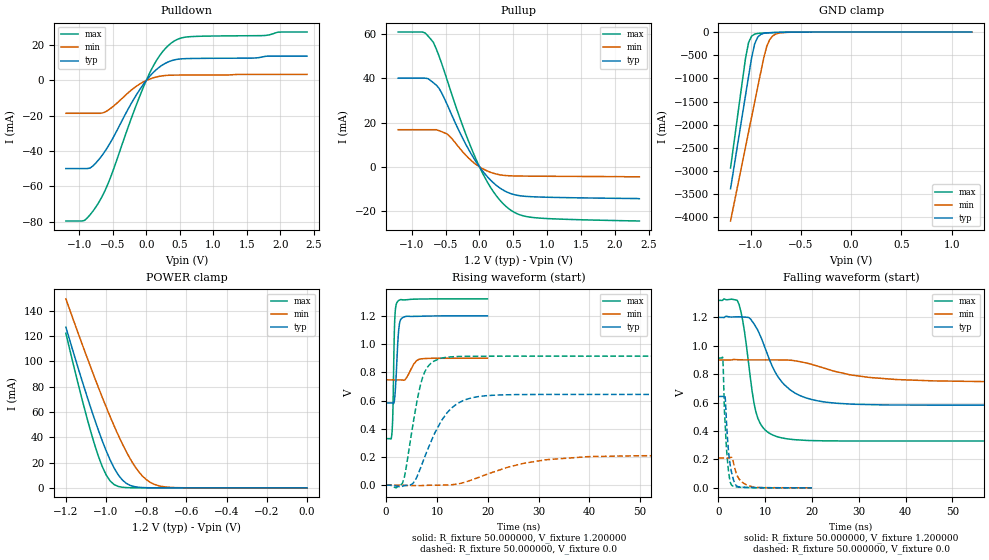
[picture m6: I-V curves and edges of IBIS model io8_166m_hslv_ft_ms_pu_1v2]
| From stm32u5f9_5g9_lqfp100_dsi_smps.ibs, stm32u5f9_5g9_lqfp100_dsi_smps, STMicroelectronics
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|   Model io8_166m_hslv_ft_ms_pu_1v2
[Model]  io8_166m_hslv_ft_ms_pu_1v2
Model_type I/O
Polarity   Non-Inverting
Enable   Active-Low
Vinl =   0.360000V
Vinh =   0.840000V
Vmeas =  0.600000V
Cref =   50.000000pF
Rref =   100.000000M
Vref =   0.0V
C_comp   3.151700pF   3.087200pF   3.197900pF
[Temperature Range]   25.000000   0.140000k   -40.000000
[Pullup Reference]   1.200000V   0.900000V   1.320000V
[Pulldown Reference]   0.0V   0.0V   0.0V
[POWER Clamp Reference]   1.200000V   0.900000V   1.320000V
[GND Clamp Reference]   0.0V   0.0V   0.0V
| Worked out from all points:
|   slope of the pulldown table from 0 to 0.18 V, typ, clamps not added: 25.4 ohm
|   slope of the pullup table from 0 to 0.18 V, typ, clamps not added: 27.8 ohm
|   GND clamp passes 1 mA (typ) near -0.51 V on its own axis
|   POWER clamp passes 1 mA (typ) near -0.86 V on its own axis
|   rising waveform, R_fixture 50.000000, V_fixture 1.200000: 20-80 % time 553ps typ, 1.42ns min, 312ps max; typ from 0.583 V to 1.2 V
|   rising waveform, R_fixture 50.000000, V_fixture 0.0: 20-80 % time 5.19ns typ, 12.1ns min, 2.72ns max; typ from 0 V to 0.643 V
|   falling waveform, R_fixture 50.000000, V_fixture 1.200000: 20-80 % time 5.91ns typ, 12.5ns min, 2.6ns max; typ from 1.2 V to 0.583 V
|   falling waveform, R_fixture 50.000000, V_fixture 0.0: 20-80 % time 1.04ns typ, 1.73ns min, 831ps max; typ from 0.643 V to 0 V
[Pulldown]
|Voltage   I(typ)   I(min)   I(max)
-1.2V     -49.86mA   -18.57mA   -79.56mA
-920mV    -49.86mA   -18.57mA   -79.19mA
-840mV    -49.6mA    -18.57mA   -76.08mA
-720mV    -45.32mA   -18.57mA   -69.74mA
-560mV    -36.71mA   -16.58mA   -57.44mA
-200mV    -11.43mA   -4.74mA    -19.03mA
0V        0A         0A         0A
160mV     6.477mA    2.075mA    11.78mA
360mV     10.99mA    2.99mA     20.81mA
480mV     12.07mA    3.054mA    23.52mA
640mV     12.43mA    3.075mA    24.76mA
2.4V      13.77mA    3.425mA    27.43mA
[Pullup]
|Voltage   I(typ)   I(min)   I(max)
-1.2V     40.07mA    16.78mA    60.91mA
-840mV    40.07mA    16.78mA    60.91mA
-680mV    37.99mA    16.78mA    56.17mA
-600mV    35.62mA    16.38mA    50.27mA
-480mV    28.32mA    14.85mA    39.45mA
-240mV    12.39mA    6.513mA    17.85mA
-40mV     1.772mA    818.2uA    2.67mA
200mV     -7.072mA   -2.851mA   -11mA
440mV     -11.84mA   -4.03mA    -19.1mA
600mV     -13.07mA   -4.154mA   -21.71mA
840mV     -13.59mA   -4.223mA   -23.04mA
2.36V     -14.4mA    -4.5mA     -24.47mA
[GND_clamp]
|Voltage   I(typ)   I(min)   I(max)
-1.2V     -3.379A    -4.076A    -2.932A
-1.05V    -1.35A     -2.47A     -550.7mA
-1.02V    -947.8mA   -2.149A    -221.5mA
-990mV    -552.4mA   -1.829A    -88.44mA
-960mV    -255.3mA   -1.51A     -44.87mA
-930mV    -111.8mA   -1.191A    -30.68mA
-870mV    -28.36mA   -564.6mA   -21.34mA
-840mV    -18.65mA   -309.5mA   -18.49mA
-810mV    -14.07mA   -161.6mA   -15.92mA
-780mV    -11.37mA   -83.33mA   -13.53mA
-600mV    -3.009mA   -4.322mA   -3.091mA
1.2V      0A         13.65nA    0A
[POWER_clamp]
|Voltage   I(typ)   I(min)   I(max)
-1.2V     127mA      149.4mA    122.2mA
-1.12V    84.98mA    114mA      70.29mA
-1.06V    55.52mA    88.42mA    35.69mA
-1.02V    37.64mA    72.04mA    17.19mA
-1V       29.52mA    64.13mA    10.33mA
-960mV    15.7mA     48.99mA    2.596mA
-900mV    3.636mA    28.77mA    207.8uA
-840mV    502.9uA    13.24mA    43.19uA
-800mV    129uA      6.535mA    43.19uA
-740mV    26.51uA    1.726mA    43.19uA
-620mV    25.02uA    82.33uA    35.3uA
0V        0A         17.36nA    0A
[Ramp]
| variable   typ   min   max
dV/dt_r  0.38571/5.18652n   0.12565/12.06910n   0.54819/2.70800n
dV/dt_f  0.37043/5.90893n   92.38800m/12.50340n 0.59405/2.58702n
R_load = 50.000000
[Rising Waveform]
R_fixture= 50.000000
V_fixture= 1.200000
V_fixture_min= 0.900000
V_fixture_max= 1.320000
|time   V(typ)   V(min)   V(max)
0s        582.6mV    746.1mV    329.9mV
1.121ns   582.8mV    746.1mV    361.9mV
1.321ns   580.5mV    746.1mV    516.1mV
1.562ns   587.1mV    746.1mV    1.006V
1.682ns   619.7mV    746.1mV    1.165V
2.282ns   1.004V     746.1mV    1.303V
2.723ns   1.161V     746.1mV    1.313V
3.644ns   1.194V     746.1mV    1.313V
6.527ns   1.197V     892.2mV    1.319V
19.94ns   1.2V       900mV      1.32V
[Rising Waveform]
R_fixture= 50.000000
V_fixture= 0.0
V_fixture_min= 0.0
V_fixture_max= 0.0
|time   V(typ)   V(min)   V(max)
0s        434.2uV    495.9uV    378.8uV
3.203ns   -7.918mV   626.1uV    14.13mV
4.004ns   -1.1mV     -2.056mV   139.1mV
5.606ns   27.97mV    -2.585mV   502.2mV
7.608ns   201.7mV    -1.561mV   803.6mV
12.01ns   513.8mV    1.518mV    906.6mV
18.42ns   628.9mV    58.36mV    913.7mV
27.23ns   642.3mV    156.1mV    914mV
40.04ns   643.2mV    202.8mV    914mV
199.4ns   643.3mV    210mV      914mV
[Falling Waveform]
R_fixture= 50.000000
V_fixture= 1.200000
V_fixture_min= 0.900000
V_fixture_max= 1.320000
|time   V(typ)   V(min)   V(max)
0s        1.2V       900mV      1.32V
4.004ns   1.204V     902.5mV    1.32V
5.205ns   1.203V     901.1mV    1.173V
7.207ns   1.173V     901mV      675.8mV
8.408ns   1.11V      901.1mV    490.8mV
11.61ns   847.5mV    901mV      372.2mV
14.41ns   716.4mV    900.2mV    346.7mV
22.82ns   604.2mV    840.6mV    331.1mV
46.05ns   582.6mV    753.2mV    329.9mV
199.4ns   582.6mV    746.1mV    329.9mV
[Falling Waveform]
R_fixture= 50.000000
V_fixture= 0.0
V_fixture_min= 0.0
V_fixture_max= 0.0
|time   V(typ)   V(min)   V(max)
0s        643.3mV    210mV      914mV
920.9ps   643.5mV    210mV      909.1mV
1.241ns   648.8mV    210.1mV    573.8mV
1.401ns   645.5mV    210.1mV    462.6mV
1.722ns   458mV      210.1mV    273.2mV
2.202ns   238.8mV    210mV      103.2mV
2.763ns   114.4mV    215.5mV    21.76mV
3.804ns   15.97mV    102.2mV    7.076mV
6.286ns   3.81mV     17.35mV    1.812mV
19.94ns   434.2uV    495.9uV    378.8uV
